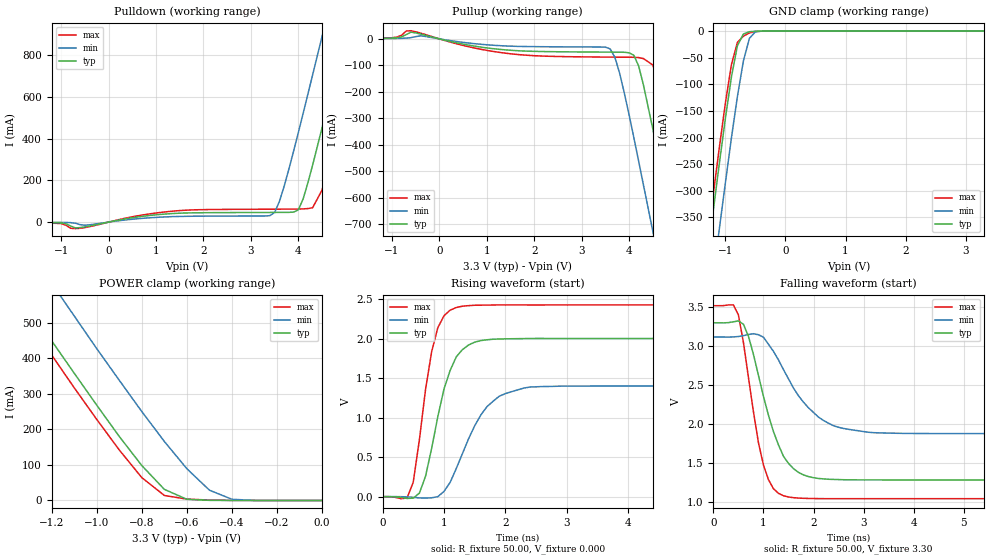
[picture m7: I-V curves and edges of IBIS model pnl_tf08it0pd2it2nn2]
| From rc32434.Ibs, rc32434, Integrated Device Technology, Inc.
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[Model]   pnl_tf08it0pd2it2nn2
Model_type   I/O
Polarity   Non-Inverting
Enable   Active-High
Vinl =  0.800V
Vinh =  2.000V
Vmeas =  1.500V
C_comp   0.40pF   0.30pF   0.50pF
[Temperature Range]   25.00   0.12k   0.000
[Voltage Range]   3.30V   3.00V   3.60V
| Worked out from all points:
|   slope of the pulldown table from 0 to 0.495 V, typ, clamps not added: 23.8 ohm
|   slope of the pullup table from 0 to 0.495 V, typ, clamps not added: 25.2 ohm
|   GND clamp passes 1 mA (typ) near -0.59 V on its own axis
|   POWER clamp passes 1 mA (typ) near -0.52 V on its own axis
|   rising waveform, R_fixture 50.00, V_fixture 0.000: 20-80 % time 362ps typ, 525ps min, 278ps max; typ from 0 V to 2 V
|   falling waveform, R_fixture 50.00, V_fixture 3.30: 20-80 % time 533ps typ, 781ps min, 372ps max; typ from 3.3 V to 1.28 V
[Pulldown]
| voltage   I(typ)   I(min)   I(max)
-3.3V     -1mA       0A         0A
-700mV    -27.7mA    -5.4mA     -31.23mA
1.3V      40.47mA    25.9mA     51.51mA
3.4V      46.38mA    31.02mA    61.99mA
3.6V      46.53mA    98.55mA    62.17mA
4V        59.07mA    430mA      62.72mA
4.3V      273mA      706mA      68.86mA
4.5V      453mA      891mA      154mA
4.9V      826mA      1.263A     506mA
5.1V      1.014A     1.449A     693mA
5.3V      1.202A     1.634A     881mA
6.6V      2.426A     2.844A     2.108A
[Pullup]
| voltage   I(typ)   I(min)   I(max)
-3.3V     1mA        1mA        1mA
-600mV    25.42mA    4.72mA     30.93mA
1.3V      -40.07mA   -25.83mA   -51.8mA
3.6V      -50mA      -37.9mA    -68.85mA
3.8V      -50.19mA   -131mA     -69.08mA
4.1V      -62.29mA   -375mA     -69.5mA
4.3V      -174mA     -552mA     -74.42mA
4.5V      -342mA     -729mA     -98.97mA
4.9V      -701mA     -1.084A    -402mA
5.1V      -882mA     -1.262A    -583mA
5.3V      -1.063A    -1.439A    -765mA
6.6V      -2.239A    -2.595A    -1.946A
[GND_clamp]
| voltage   I(typ)   I(min)   I(max)
-3.3V     -2.234A    -2.325A    -2.213A
-1.3V     -425mA     -548mA     -395mA
-1.2V     -336mA     -459mA     -305mA
-1.1V     -248mA     -371mA     -218mA
-1V       -164mA     -285mA     -135mA
-900mV    -86.4mA    -201mA     -63.27mA
-800mV    -27.52mA   -123mA     -21.14mA
-700mV    -5.277mA   -55.94mA   -9.346mA
-600mV    -1.092mA   -13.46mA   -3.426mA
-500mV    -154uA     -1.295mA   -660uA
-300mV    -13.82uA   -13.04uA   -19.46uA
3.3V      49.8uA     220uA      75.12uA
[POWER_clamp]
| voltage   I(typ)   I(min)   I(max)
-3.3V     2.423A     2.563A     2.388A
-1.4V     636mA      796mA      595mA
-1.3V     542mA      703mA      502mA
-1.2V     449mA      611mA      409mA
-1.1V     358mA      519mA      317mA
-900mV    180mA      338mA      142mA
-800mV    98.21mA    250mA      64.3mA
-700mV    31.26mA    166mA      14.09mA
-600mV    3.334mA    89.25mA    3.864mA
-500mV    425uA      29.04mA    1.253mA
-400mV    34.58uA    3.355mA    239uA
0V        0A         0A         0A
[Ramp]
| variable   typ   min   max
dV/dt_r   1.20/0.36n   0.84/0.53n   1.46/0.28n
dV/dt_f   1.21/0.53n   0.83/0.78n   1.46/0.39n
R_load = 50.00
[Rising Waveform]
R_fixture = 50.00
V_fixture = 0.000
| time   V(typ)   V(min)   V(max)
0s        0V         554nV      0V
400ps     -22.93mV   -3.213mV   -17.45mV
500ps     -18.63mV   -8.865mV   184mV
600ps     44.48mV    -16.41mV   720mV
800ps     614mV      -14.59mV   1.837V
900ps     1.013V     -209uV     2.138V
1.2ns     1.769V     356mV      2.393V
1.7ns     1.985V     1.139V     2.424V
2.4ns     2.001V     1.387V     2.425V
9.9ns     2.001V     1.4V       2.426V
[Falling Waveform]
R_fixture = 50.00
V_fixture = 3.30
| time   V(typ)   V(min)   V(max)
0s        3.299V     3.117V     3.518V
400ps     3.312V     3.118V     3.528V
500ps     3.323V     3.123V     3.401V
700ps     3.127V     3.149V     2.601V
1ns       2.357V     3.115V     1.477V
1.2ns     1.905V     2.933V     1.173V
1.4ns     1.588V     2.699V     1.083V
2.1ns     1.304V     2.09V      1.046V
2.8ns     1.287V     1.924V     1.045V
9.9ns     1.285V     1.879V     1.045V
